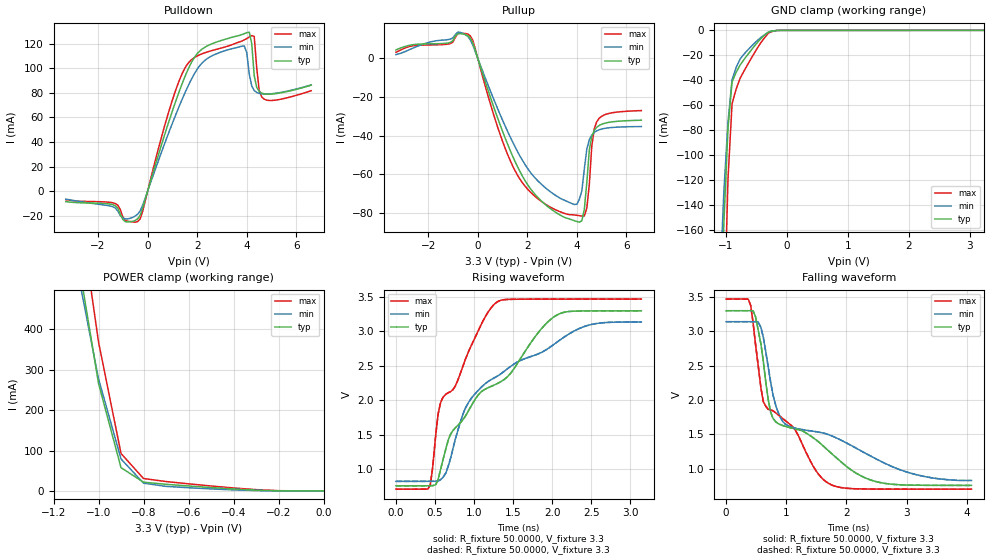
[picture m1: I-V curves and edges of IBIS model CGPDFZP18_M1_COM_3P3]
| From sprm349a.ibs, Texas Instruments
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|   Model Cell CGPDFZP18_M1_COM_3P3
[Model]   CGPDFZP18_M1_COM_3P3
Model_type   I/O
Polarity   Non-Inverting
Enable   Active-Low
Vinl =  0.8
Vinh =  2.0
Cref =  10.0000pF
Rref =  50.0000
Vref =  1.5V
Vmeas =  1.5
C_comp   2.231182p   2.070767p   2.288404p
[Temperature Range]   25   105   0
[Voltage Range]   3.3   3.14   3.47
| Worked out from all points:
|   slope of the pulldown table from 0 to 0.495 V, typ, clamps not added: 14.8 ohm
|   slope of the pullup table from 0 to 0.495 V, typ, clamps not added: 25.3 ohm
|   GND clamp passes 1 mA (typ) near -0.28 V on its own axis
|   POWER clamp passes 1 mA (typ) near -0.24 V on its own axis
|   rising waveform, R_fixture 50.0000, V_fixture 3.3: 20-80 % time 1.07ns typ, 1.09ns min, 526ps max; typ from 0.759 V to 3.3 V
|   rising waveform, R_fixture 50.0000, V_fixture 3.3: 20-80 % time 1.07ns typ, 1.09ns min, 526ps max; typ from 0.759 V to 3.3 V
|   falling waveform, R_fixture 50.0000, V_fixture 3.3: 20-80 % time 1.11ns typ, 1.51ns min, 844ps max; typ from 3.3 V to 0.756 V
|   falling waveform, R_fixture 50.0000, V_fixture 3.3: 20-80 % time 1.11ns typ, 1.51ns min, 844ps max; typ from 3.3 V to 0.756 V
[POWER_clamp]
|   voltage   I(typ)   I(min)   I(max)
-3.3V     9.989A     8.641A     10.98A
-1.1V     604.7mA    564.8mA    757.9mA
-1.067V   491.9mA    469.1mA    628.2mA
-1.033V   379mA      373.4mA    498.6mA
-1V       266.2mA    277.7mA    368.9mA
-900mV    57.62mA    79.25mA    92.72mA
-800mV    21.66mA    19.3mA     30.71mA
-700mV    16.38mA    11.26mA    23.26mA
-300mV    1.929mA    789.7uA    3.217mA
-200mV    292.8uA    98.01uA    616uA
-11.55fV  2.899uA    2.516uA    6.987uA
[Pulldown]
|   voltage   I(typ)   I(min)   I(max)
-3.3V     -8.456mA   -6.412mA   -6.88mA
-1.4V     -10.96mA   -12.65mA   -9.431mA
-400mV    -22.4mA    -18.63mA   -24.71mA
1.3V      82.47mA    70.34mA    91.21mA
1.9V      109.2mA    95.96mA    108.8mA
2.5V      119.1mA    109mA      113.8mA
3.9V      128.1mA    118.1mA    123mA
4.1V      129.4mA    95.25mA    125.3mA
4.3V      94.03mA    81.92mA    125.9mA
4.5V      81.16mA    79.48mA    82.05mA
4.7V      79.16mA    78.96mA    74.86mA
6.6V      86.26mA    86.47mA    81.73mA
[Pullup]
|   voltage   I(typ)   I(min)   I(max)
-3.3V     4.286mA    1.847mA    3.065mA
-800mV    12.73mA    13.5mA     12.77mA
-300mV    10.41mA    9.538mA    11.56mA
1.5V      -53.19mA   -45.63mA   -57.95mA
2.4V      -71.6mA    -63.02mA   -72.32mA
3.6V      -82.66mA   -73.95mA   -80.54mA
4V        -84.35mA   -75.4mA    -81.13mA
4.3V      -77.99mA   -57.15mA   -81.46mA
4.5V      -47.49mA   -42.07mA   -65.42mA
4.6V      -40.38mA   -39.67mA   -45.57mA
4.7V      -37.3mA    -38.33mA   -36.43mA
6.6V      -32.02mA   -35.3mA    -27.05mA
[GND_clamp]
|   voltage   I(typ)   I(min)   I(max)
-3.3V     -13.5A     -11.63A    -14.67A
-1.1V     -264.6mA   -203.9mA   -420.9mA
-1.033V   -153.2mA   -128.2mA   -239.9mA
-966.7mV  -78.76mA   -73.45mA   -119.2mA
-900mV    -41.29mA   -39.54mA   -58.78mA
-833.3mV  -33.75mA   -29.74mA   -47.13mA
-766.7mV  -27.7mA    -22.83mA   -38.28mA
-500mV    -10.62mA   -8.784mA   -15.38mA
-300mV    -1.267mA   -1.441mA   -2.149mA
-166.7mV  -65.92uA   -134.5uA   -140.6uA
-100mV    -13.31uA   -16.6uA    -57.02uA
3.233V    2.695uA    14.19uA    5.948uA
[Ramp]
| variable   typ   min   max
dV/dt_f   1.527004/1.114204n   1.396478/1.538716n   1.661303/0.8437641n
dV/dt_r   1.294871/1.220033n   1.170741/1.321146n   1.424292/0.6794892n
R_load = 50
[Rising Waveform]
R_fixture = 50.0000
V_fixture = 3.3
V_fixture_min = 3.14
V_fixture_max = 3.47
|   time   V(typ)   V(min)   V(max)
0s        759.5mV    824.1mV    710.6mV
440ps     760.6mV    824.5mV    773.5mV
540ps     853.3mV    830.3mV    1.802V
570ps     990.2mV    847.7mV    1.961V
700ps     1.509V     1.162V     2.127V
890ps     1.773V     1.889V     2.599V
1.28ns    2.234V     2.34V      3.415V
2.09ns    3.254V     2.869V     3.469V
2.51ns    3.298V     3.103V     3.469V
3.14ns    3.299V     3.137V     3.47V
[Rising Waveform]
R_fixture = 50.0000
V_fixture = 3.3
V_fixture_min = 3.14
V_fixture_max = 3.47
|   time   V(typ)   V(min)   V(max)
0s        759.5mV    824.1mV    710.6mV
440ps     760.6mV    824.5mV    773.5mV
540ps     853.3mV    830.3mV    1.802V
570ps     990.2mV    847.7mV    1.961V
700ps     1.509V     1.162V     2.127V
890ps     1.773V     1.889V     2.599V
1.28ns    2.234V     2.34V      3.415V
2.09ns    3.254V     2.869V     3.469V
2.51ns    3.298V     3.103V     3.469V
3.14ns    3.299V     3.137V     3.47V
[Falling Waveform]
R_fixture = 50.0000
V_fixture = 3.3
V_fixture_min = 3.14
V_fixture_max = 3.47
|   time   V(typ)   V(min)   V(max)
0s        3.3V       3.14V      3.47V
370ps     3.3V       3.14V      3.469V
450ps     3.297V     3.14V      3.123V
620ps     2.561V     2.912V     1.973V
700ps     2.011V     2.487V     1.864V
780ps     1.733V     2.078V     1.843V
990ps     1.614V     1.646V     1.695V
1.66ns    1.295V     1.508V     811.5mV
2.5ns     809.8mV    1.139V     702.5mV
4.08ns    755.8mV    827.8mV    701.2mV
[Falling Waveform]
R_fixture = 50.0000
V_fixture = 3.3
V_fixture_min = 3.14
V_fixture_max = 3.47
|   time   V(typ)   V(min)   V(max)
0s        3.3V       3.14V      3.47V
370ps     3.3V       3.14V      3.469V
450ps     3.297V     3.14V      3.123V
620ps     2.561V     2.912V     1.973V
700ps     2.011V     2.487V     1.864V
780ps     1.733V     2.078V     1.843V
990ps     1.614V     1.646V     1.695V
1.66ns    1.295V     1.508V     811.5mV
2.5ns     809.8mV    1.139V     702.5mV
4.08ns    755.8mV    827.8mV    701.2mV
